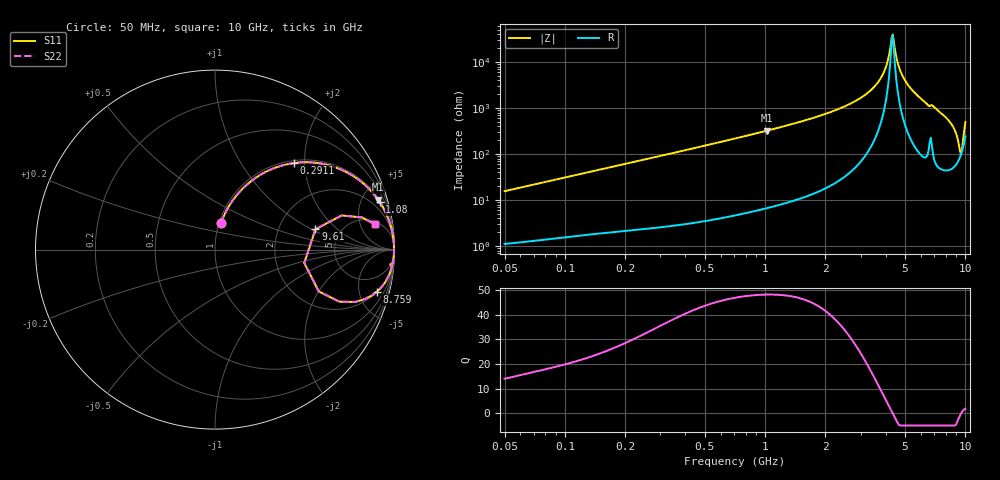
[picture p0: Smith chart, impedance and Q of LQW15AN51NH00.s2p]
!Murata Part Number: LQW15AN51NH00
!These Parameters are Measured in Series Mode Connection
!  o--[Z]--o
!Port1  Port2
!  o-------o
!Freq. Start=50[MHz] Stop=10[GHz], 401[Steps]
# Hz S RI R 50
!Freq.(Hz)	S 11(Real)	S 11(Imag)	S 21(Real)	S 21(Imag)	S 12(Real)	S 12(Imag)	S 22(Real)	S 22(Imag)
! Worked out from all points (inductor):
!   401 points, 50 MHz to 10 GHz, reference 50 ohm
!   read as one part in series: L = 49.6 nH near 51.34 MHz
!   highest Q = 48.2 at 1.025 GHz (marker M1), where L = 50.4 nH
!   self-resonance near 4.284 GHz
!   S11 on the Smith chart (normalised r, x): 50 MHz: 1.02, +0.31; 291.1 MHz: 1.05, +1.77; 1.08 GHz: 1.14, +6.88; 8.759 GHz: 2.04, -7.20; 9.61 GHz: 3.26, +1.09; 10 GHz: 6, +9
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5e7  0.0342 0.1493  0.9658 -0.1493  0.9658 -0.1493  0.0342 0.1493
1.214486e8  0.1337 0.3181  0.8663 -0.3181  0.8663 -0.3181  0.1337 0.3181
2.911136e8  0.4416 0.4825  0.5584 -0.4825  0.5584 -0.4825  0.4416 0.4825
2.949953e8  0.4479 0.4833  0.5521 -0.4833  0.5521 -0.4833  0.4479 0.4833
7.071068e8  0.8212 0.3727  0.1788 -0.3727  0.1788 -0.3727  0.8212 0.3727
1.024606e9  0.9084 0.2783  0.0916 -0.2783  0.0916 -0.2783  0.9084 0.2783
1.080357e9  0.9174 0.2651  0.0826 -0.2651  0.0826 -0.2651  0.9174 0.2651
1.717543e9  0.9698 0.1603  0.0302 -0.1603  0.0302 -0.1603  0.9698 0.1603
2.555552e9  0.9898 0.0864  0.0102 -0.0864  0.0102 -0.0864  0.9898 0.0864
3.286879e9  0.9956 0.0446  0.00439 -0.0446  0.00439 -0.0446  0.9956 0.0446
3.853138e9  0.9973 0.019  0.00273 -0.019  0.00273 -0.019  0.9973 0.019
4.009335e9  0.9975 0.0125  0.00254 -0.0125  0.00254 -0.0125  0.9975 0.0125
4.171863e9  0.9976 0.00601  0.00244 -0.00601  0.00244 -0.00601  0.9976 0.00601
4.283859e9  0.9976 0.00163  0.00243 -0.00163  0.00243 -0.00163  0.9976 0.00163
4.34098e9  0.9976 -0.000576  0.00244 0.000576  0.00244 0.000576  0.9976 -0.000576
4.700058e9  0.9972 -0.0141  0.00275 0.0141  0.00275 0.0141  0.9972 -0.0141
5.156693e9  0.9963 -0.0306  0.00372 0.0306  0.00372 0.0306  0.9963 -0.0306
7.878683e9  0.9683 -0.1447  0.0317 0.1447  0.0317 0.1447  0.9683 -0.1447
8.759398e9  0.9004 -0.2359  0.0996 0.2359  0.0996 0.2359  0.9004 -0.2359
9.236013e9  0.6936 -0.2903  0.3064 0.2903  0.3064 0.2903  0.6936 -0.2903
9.610418e9  0.5594 0.1129  0.4406 -0.1129  0.4406 -0.1129  0.5594 0.1129
1e10  0.8888 0.1416  0.1112 -0.1416  0.1112 -0.1416  0.8888 0.1416
